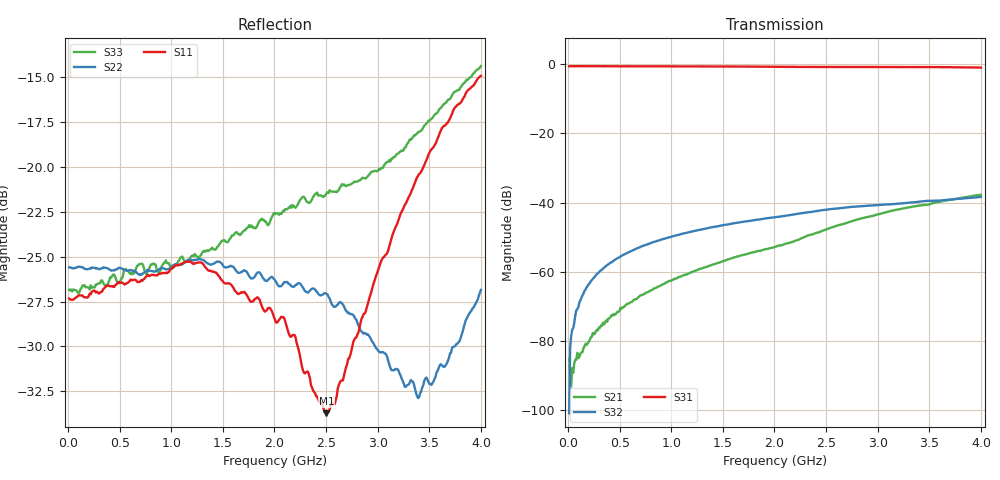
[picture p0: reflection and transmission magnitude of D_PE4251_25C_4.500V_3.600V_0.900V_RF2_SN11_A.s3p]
! Device ID: PE4251_SoldCshunt_081809
! Dir: c:\Test Bench Repositories\Bench_Software_CVI_Version_8\trunk\PSC 4Port_VNA Bench\datalog\4250\TEST\PE4251_SoldCshunt_081809\25C\4p500000\RF2
! Serial: 11
! Insertion: A
! Temp: 25C
! VDD: 4.500
! Control_Hi: 80.000
! Control_Lo: 20.000
! Logic State: RF2
! Port 1: RFC
! Port 2: RF1
! Port 3: RF2
! V1 = 0.90
! V2 = 0.90
! V3 = 0.90
! IDD: 5.788670e-05
! FILE NAME
! DATE 08/18/09  20:14
! CORRECTED  DATA
#  Hz  S  RI  R  50.00
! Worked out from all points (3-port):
!   401 points, 10 MHz to 4 GHz, reference 50 ohm
!   strongest paths, dB at 10 MHz, 1.008 GHz, 2.005 GHz, 3.002 GHz, 4 GHz:
!     S31: -0.6, -0.6, -0.7, -0.7, -1.0
!     S32: -100.9, -49.8, -44.2, -40.7, -38.3
!     S21: -85.2, -62.4, -52.8, -43.4, -37.7
!   lowest |S11| = -33.7 dB at 2.504 GHz (marker M1), VSWR 1.04, Z = 50.5 - j2.01 ohm
!   |S11| at or under -10 dB: start of sweep to end of sweep
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1e7  0.043 -0.000655  4.85e-05 -1.61e-05  0.9378 -0.00305
     3.23e-05 4.49e-05  0.0525 -0.000914  6.44e-05 8.24e-05
     0.9381 -0.00517  -5.93e-06 -6.78e-06  0.0455 0.000381
9.9775e7  0.0438 0.00143  1.23e-05 -5.4e-05  0.9382 -0.0357
          1.18e-05 -5.52e-05  0.0527 -0.000956  4.31e-05 0.000318
          0.939 -0.0354  3.81e-05 0.000307  0.0444 -0.000169
1.79575e8  0.0432 0.00221  -3.53e-06 -0.000107  0.9362 -0.0633
           5.09e-06 -8.76e-05  0.0518 -0.00127  5e-05 0.000587
           0.9368 -0.0632  4.7e-05 0.000598  0.0462 0.000731
2.99275e8  0.0443 0.00291  -4.77e-05 -0.000149  0.9321 -0.1046
           -4.24e-05 -0.000151  0.0517 -0.00251  7.63e-05 0.000982
           0.9321 -0.1043  8.28e-05 0.000981  0.0473 -0.000848
4.98775e8  0.0476 0.00122  -0.000168 -0.000224  0.9199 -0.171
           -0.000164 -0.000216  0.0521 -0.00456  0.000156 0.00163
           0.9202 -0.1712  0.000153 0.00163  0.0473 -0.00403
1.0873e9  0.0523 -0.0112  -0.000796 -0.000323  0.8608 -0.3582
          -0.000788 -0.000328  0.0519 -0.0118  0.000507 0.00345
          0.862 -0.3581  0.000514 0.00345  0.0547 -0.011
2.005e9  0.0349 -0.0137  -0.00225 -0.000424  0.6975 -0.6028
         -0.00225 -0.00043  0.0479 -0.00685  0.00115 0.00604
         0.6989 -0.6023  0.00115 0.00607  0.0666 -0.0316
2.50375e9  0.0056 -0.0198  -0.00402 -0.000842  0.5869 -0.7
           -0.00403 -0.000853  0.0443 0.000265  0.00157 0.00776
           0.5893 -0.6999  0.00156 0.00776  0.0532 -0.0652
3.391525e9  -0.0861 -0.0384  -0.009 0.000971  0.35 -0.8432
            -0.00896 0.000978  0.0132 0.0185  0.00227 0.00999
            0.3515 -0.8436  0.00224 0.01  -0.0259 -0.122
4e9  -0.1767 -0.0268  -0.0126 0.00359  0.1357 -0.8867
     -0.0125 0.00357  -0.0265 0.0369  0.00238 0.0118
     0.1374 -0.8852  0.00238 0.0119  -0.1328 -0.1362
